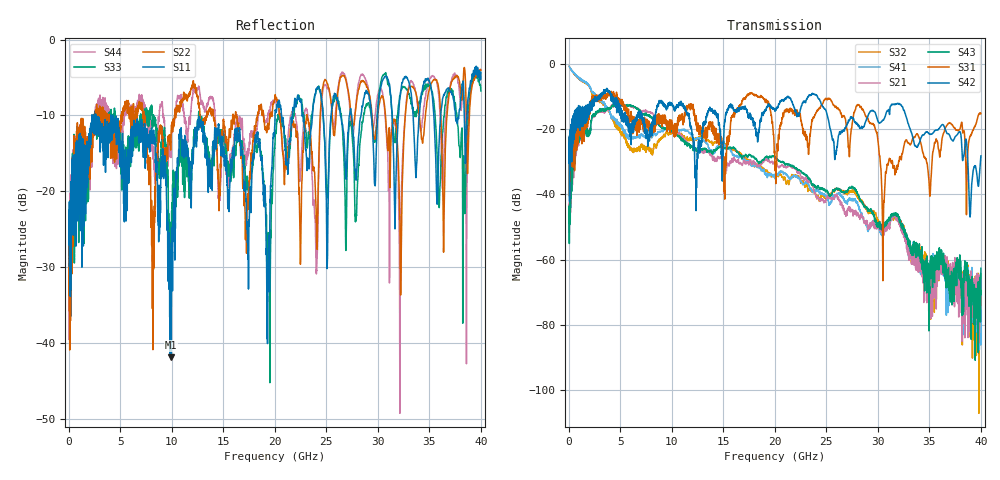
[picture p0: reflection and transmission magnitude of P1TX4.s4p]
!Agilent Technologies,N5245A,MY49151084,A.09.20.08
!Agilent N5245A: A.09.20.08
!Date: Thursday, March 01, 2012 10:51:05
!Correction: S11(Full 4 Port(1,2,3,4))
!S12(Full 4 Port(1,2,3,4))
!S13(Full 4 Port(1,2,3,4))
!S14(Full 4 Port(1,2,3,4))
!S21(Full 4 Port(1,2,3,4))
!S22(Full 4 Port(1,2,3,4))
!S23(Full 4 Port(1,2,3,4))
!S24(Full 4 Port(1,2,3,4))
!S31(Full 4 Port(1,2,3,4))
!S32(Full 4 Port(1,2,3,4))
!S33(Full 4 Port(1,2,3,4))
!S34(Full 4 Port(1,2,3,4))
!S41(Full 4 Port(1,2,3,4))
!S42(Full 4 Port(1,2,3,4))
!S43(Full 4 Port(1,2,3,4))
!S44(Full 4 Port(1,2,3,4))
!S4P File: Measurements: <S11,S12,S13,S14>,
!<S21,S22,S23,S24>,
!<S31,S32,S33,S34>,
!<S41,S42,S43,S44>:
# Hz S  dB  R 50
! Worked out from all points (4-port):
!   3996 points, 50 MHz to 40 GHz, reference 50 ohm
!   strongest paths, dB at 50 MHz, 10.04 GHz, 20.03 GHz, 30.02 GHz, 40 GHz:
!     S42: -26.6, -12.6, -14.5, -17.6, -28.2
!     S31: -26.4, -19.1, -31.1, -23.9, -15.3
!     S43: -48.3, -20.9, -28.6, -49.3, -62.6
!     S21: -46.7, -20.0, -31.0, -49.8, -73.8
!     S41: -0.7, -19.7, -34.9, -50.1, -67.5
!     S32: -0.8, -20.7, -34.4, -48.4, -68.4
!   lowest |S11| = -41.9 dB at 9.92 GHz (marker M1), VSWR 1.02, Z = 49.2 + j0.25 ohm
!   |S11| at or under -10 dB: start of sweep to 2.263 GHz; 2.64 GHz to 4.109 GHz (1.469 GHz wide, 43.5 % of centre); 4.33 GHz to 20.03 GHz (15.7 GHz wide, 129 % of centre)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
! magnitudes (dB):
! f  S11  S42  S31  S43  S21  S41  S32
! 50 MHz  -24.0  -26.6  -26.4  -48.3  -46.7  -0.7  -0.8
! 2.79 GHz  -10.2  -10.2  -10.0  -14.6  -14.8  -10.3  -10.8
! 9.92 GHz  -41.9  -12.2  -18.5  -20.3  -19.5  -19.8  -21.3
! 24.01 GHz  -6.5  -9.5  -15.0  -37.8  -40.5  -39.1  -40.6
! 28.17 GHz  -12.4  -19.1  -12.6  -40.6  -46.4  -44.2  -41.4
! 30.53 GHz  -5.2  -17.3  -50.7  -49.8  -51.3  -51.3  -51.6
! 40 GHz  -5.2  -28.2  -15.3  -62.6  -73.8  -67.5  -68.4
